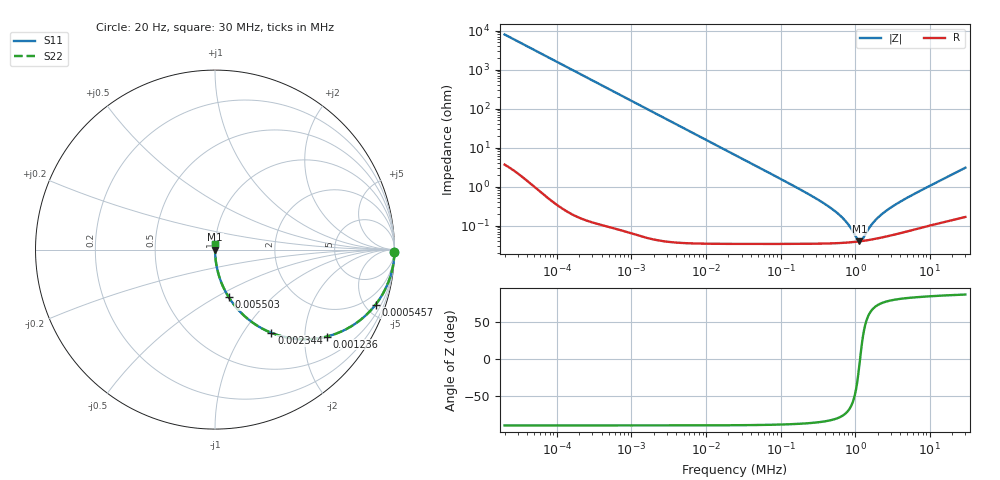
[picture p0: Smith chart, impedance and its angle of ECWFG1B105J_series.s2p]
!  *** S-Parameter ***
!  Copyright (C) Panasonic Industry
!  Plastic Film Capacitor (ECWFG)
!  Parts No. ECWFG1B105J
!  Connection Mode : Series
!  1  o---||---o  2
!  GND o--------o GND
!  Conditions : Temperature = 20   DC Bias = 0 V
! Frequency Range : 20 Hz  -  30 MHz  [ 401 Steps ]
# Hz S RI R 50
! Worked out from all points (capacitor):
!   401 points, 20 Hz to 30 MHz, reference 50 ohm
!   read as one part in series: C = 1 uF near 21.47 Hz
!   lowest |Z| = 39.9 mohm at 1.139 MHz (marker M1)
!   series resonance near 1.163 MHz, so ESL is about 19 nH
!   S11 on the Smith chart (normalised r, x): 20 Hz: open; 545.7 Hz: 1.00, -5.82; 1.236 kHz: 1.00, -2.57; 2.344 kHz: 1.00, -1.35; 5.503 kHz: 1.00, -0.58; 30 MHz: 1.00, +0.06
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20  0.9998 -0.0126  0.000165 0.0126  0.000165 0.0126  0.9998 -0.0126
80.02006  0.9975 -0.0503  0.00255 0.0503  0.00255 0.0503  0.9975 -0.0503
216.5336  0.9817 -0.1339  0.0183 0.1339  0.0183 0.1339  0.9817 -0.1339
545.7217  0.8942 -0.3074  0.1058 0.3074  0.1058 0.3074  0.8942 -0.3074
806.8889  0.7946 -0.4038  0.2054 0.4038  0.2054 0.4038  0.7946 -0.4038
1236.222  0.6225 -0.4845  0.3775 0.4845  0.3775 0.4845  0.6225 -0.4845
2344.34  0.3146 -0.464  0.6854 0.464  0.6854 0.464  0.3146 -0.464
3591.727  0.1637 -0.3696  0.8363 0.3696  0.8363 0.3696  0.1637 -0.3696
5502.829  0.0771 -0.2662  0.9229 0.2662  0.9229 0.2662  0.0771 -0.2662
11204.45  0.02 -0.1388  0.98 0.1388  0.98 0.1388  0.02 -0.1388
24494.9  0.00452 -0.0645  0.9955 0.0645  0.9955 0.0645  0.00452 -0.0645
265198.4  0.000375 -0.00567  0.9996 0.00567  0.9996 0.00567  0.000375 -0.00567
452037.4  0.000358 -0.00297  0.9996 0.00297  0.9996 0.00297  0.000358 -0.00297
645025.1  0.000362 -0.00169  0.9996 0.00169  0.9996 0.00169  0.000362 -0.00169
798395.3  0.00037 -0.00104  0.9996 0.00104  0.9996 0.00104  0.00037 -0.00104
1061060  0.000388 -0.000247  0.9996 0.000247  0.9996 0.000247  0.000388 -0.000247
1139253  0.000395 -5.51e-05  0.9996 5.51e-05  0.9996 5.51e-05  0.000395 -5.51e-05
1267480  0.000406 0.000232  0.9996 -0.000232  0.9996 -0.000232  0.000406 0.000232
1874060  0.000462 0.00131  0.9995 -0.00131  0.9995 -0.00131  0.000462 0.00131
2871218  0.000555 0.00269  0.9994 -0.00269  0.9994 -0.00269  0.000555 0.00269
6276987  0.000839 0.00653  0.9992 -0.00653  0.9992 -0.00653  0.000839 0.00653
3e7  0.00259 0.0303  0.9974 -0.0303  0.9974 -0.0303  0.00259 0.0303
